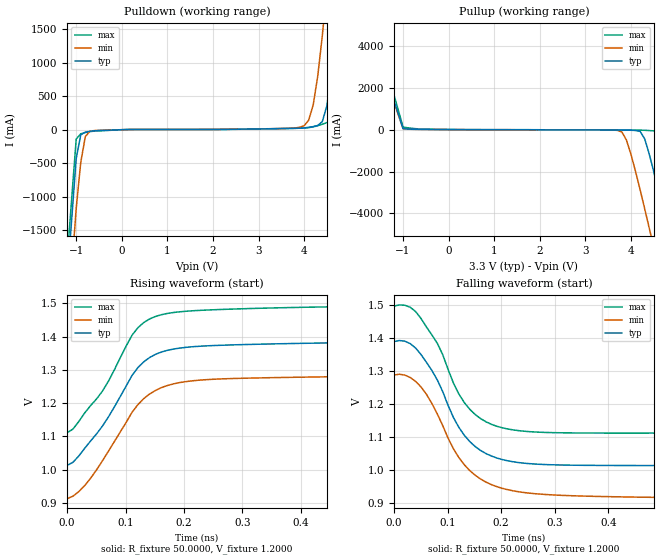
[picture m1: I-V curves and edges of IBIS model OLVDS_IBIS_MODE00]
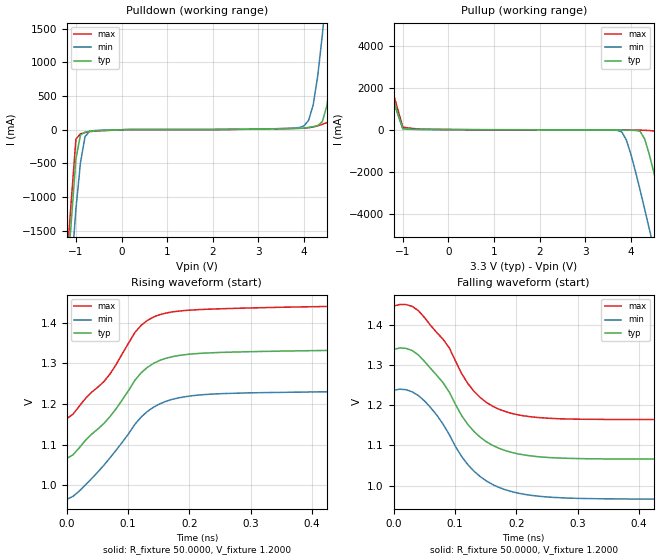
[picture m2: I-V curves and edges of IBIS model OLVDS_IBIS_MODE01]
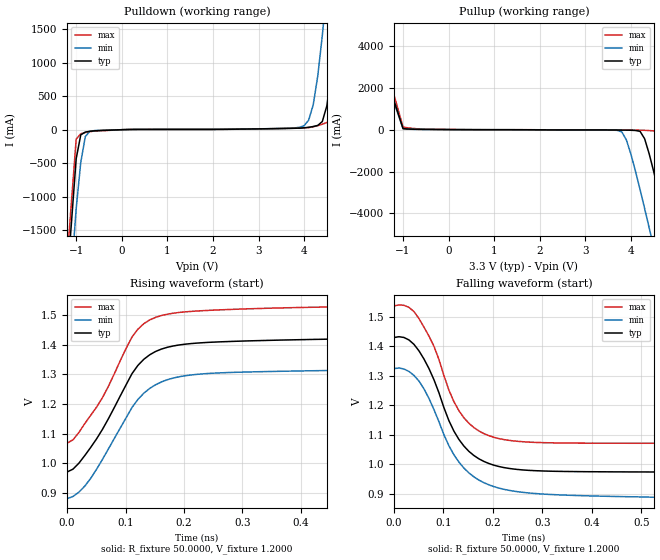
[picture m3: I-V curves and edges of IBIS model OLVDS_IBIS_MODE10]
| modified package RLC table on Oct 18th
| IBIS file olvds_ibis.ibs created by s2ibis2 version 1.1
| North Carolina State University Electronics Research Laboratory  1995
[IBIS ver]   3.2
[File name]   olvds_ibis.ibs
[File Rev]   1.0
[Date]   Oct 18, 2004
[Source]   Data created at Wipro Technologies
[Notes]   GS30 LVDS Driver
[Disclaimer] Please be aware that in the absence of a written agreement,
   Texas Instruments (TI) assumes no liability for: 1) the
   accuracy of the IBIS models provided to your company, 2) the
   proper functioning of these IBIS models in your design or for
   any resulting applications, or; 3) infringement of patents,
   copyrights, or intellectual property rights resulting from
   your use of these IBIS models. TI provides IBIS models as a
   service to our customers and therefore reserves the right to
   limit distribution of the IBIS models.
[Copyright]   Property of Texas Instruments Incorporated. Unauthorized
   reproduction and/or distribution is strictly prohibited. This
   product is protected under copyright law and trade secret law
   as an unpublished work. Copyright (C) 2003, Texas Instruments
   Incorporated, all rights reserved. These commodities are under
   the U.S. Government distribution license control. As such,
   they are not to be re-exported without the prior approval of
   the U.S. Department of Commerce.
|   Component OLVDS_IBIS
[Component]   OLVDS_IBIS
[Manufacturer]   Texas Instruments.
[Package]
| variable   typ   min   max
R_pkg   0.2   0.2   0.2
L_pkg   3.1nH   1.5nH   5.0nH
C_pkg   2.4pF   1.8pF   3.1pF
[Pin]  signal_name   model_name   R_pin   L_pin   C_pin
1   AVDD   POWER
|2   INP1   dummy
|3   INM1   dummy
4   AVSS   GND
|5   INP2   dummy
|6   INM2   dummy
7   AVDD   POWER
8   AVSS   GND
|9   INP3   dummy
|10   INM3   dummy
11   AVSS   GND
|12   INP4   dummy
|13   INM4   dummy
14   AVDD   POWER
15   LVSS   GND
|16   PD   dummy
17   LVSS   GND
18   LVSS   GND
19   LCLKP   OPERATIONAL_MODE
20   LCLKM   OPERATIONAL_MODE
21   OUTP1   OPERATIONAL_MODE
22   OUTM1   OPERATIONAL_MODE
23   OUTP2   OPERATIONAL_MODE
24   OUTM2   OPERATIONAL_MODE
25   LVDD   POWER
26   LVSS   GND
27   OUTP3   OPERATIONAL_MODE
28   OUTM3   OPERATIONAL_MODE
29   OUTP4   OPERATIONAL_MODE
30   OUTM4   OPERATIONAL_MODE
31   OUTP5   OPERATIONAL_MODE
32   OUTM5   OPERATIONAL_MODE
33   OUTP6   OPERATIONAL_MODE
34   OUTM6   OPERATIONAL_MODE
35   LVDD   POWER
36   LVSS   GND
37   OUTP7   OPERATIONAL_MODE
38   OUTM7   OPERATIONAL_MODE
39   OUTP8   OPERATIONAL_MODE
40   OUTM8   OPERATIONAL_MODE
41   ADCLKP   OPERATIONAL_MODE
42   ADCLKM   OPERATIONAL_MODE
43   LVSS   GND
44   LVSS   GND
|45   RESETZ   dummy
46   LVSS   GND
47   AVDD   POWER
|48   INP5   dummy
|49   INM5   dummy
50   AVSS   GND
|51   INP6   dummy
|52   INM6   dummy
53   AVSS   GND
54   AVDD   POWER
|55   INP7   dummy
|56   INM7   dummy
57   AVSS   GND
|58   INP8   dummy
|59   INM8   dummy
60   AVDD   POWER
61   AVSS   GND
62   AVSS   GND
63   AVDD   POWER
|64   ISET   dummy
|65   VCM   dummy
|66   REFM   dummy
|67   REFP   dummy
68   AVSS   GND
|69   INT   dummy
70   AVDD   POWER
|71   ADCLK   dummy
72   AVSS   GND
73   AVSS   GND
74   AVSS   GND
75   AVDD   POWER
|76   CSZ   dummy
|77   SDA   dummy
|78   SCLK   dummy
79   AVSS   GND
80   AVSS   GND
[Diff Pin]   inv_pin   vdiff   tdelay_typ   tdelay_min   tdelay_max
19   20   350mV   0   0   0
21   22   350mV   0   0   0
23   24   350mV   0   0   0
27   28   350mV   0   0   0
29   30   350mV   0   0   0
31   32   350mV   0   0   0
33   34   350mV   0   0   0
37   38   350mV   0   0   0
39   40   350mV   0   0   0
41   42   350mV   0   0   0
[Model Selector]   OPERATIONAL_MODE
OLVDS_IBIS_MODE00   Cell with  current setting of 3.5mA
OLVDS_IBIS_MODE01   Cell with  current setting of 2.5mA
OLVDS_IBIS_MODE10   Cell with  current setting of 4.5mA
OLVDS_IBIS_MODE11   Cell with  current setting of 6.0mA
| Models and submodels in the file (4): OLVDS_IBIS_MODE00 (Output), OLVDS_IBIS_MODE01 (Output), OLVDS_IBIS_MODE10 (Output), OLVDS_IBIS_MODE11 (Output)
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|   Model OLVDS_IBIS_MODE00
[Model]   OLVDS_IBIS_MODE00
Model_type   Output
Polarity   Inverting
Vmeas =   1.2000V
Cref =   5.0000pF
Rref = 50.0000
Vref =   1.2000V
C_comp   2.0000pF   1.5000pF   2.5000pF
[Temperature Range]   25.0000   0.1250k   -40.0000
[Voltage Range]   3.3000V   3.0000V   3.6000V
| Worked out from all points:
|   slope of the pulldown table from 0 to 0.495 V, typ, clamps not added: 131 ohm
|   slope of the pullup table from 0 to 0.495 V, typ, clamps not added: 106 ohm
|   rising waveform, R_fixture 50.0000, V_fixture 1.2000: 20-80 % time 83.5ps typ, 84.2ps min, 79.4ps max; typ from 1.01 V to 1.39 V
|   falling waveform, R_fixture 50.0000, V_fixture 1.2000: 20-80 % time 74.4ps typ, 82.1ps min, 72.4ps max; typ from 1.39 V to 1.01 V
[Pulldown]
| voltage   I(typ)   I(min)   I(max)
-3.3V     -22.38A    -23.14A    -21.96A
-2V       -9.6A      -10.42A    -9.138A
-1V       -431.5mA   -1.175A    -140.1mA
-900mV    -77.67mA   -488.8mA   -60.72mA
-800mV    -35.24mA   -102.6mA   -42.54mA
4V        27.23mA    59.11mA    24.41mA
4.2V      46.48mA    369mA      42.24mA
4.4V      121mA      1.402A     81.02mA
4.5V      356.5mA    2.114A     106.7mA
4.7V      1.539A     3.721A     310.2mA
4.9V      3.159A     5.456A     1.534A
6.6V      19.22A     21.51A     17.53A
[Pullup]
| voltage   I(typ)   I(min)   I(max)
-3.3V     19.22A     18.61A     20.47A
-2V       6.763A     6.35A      7.855A
-1V       50.05mA    51.47mA    127mA
3.8V      -16.47mA   -107.5mA   -13.35mA
4V        -25.62mA   -1.176A    -16.52mA
4.3V      -431.6mA   -3.769A    -27.64mA
4.4V      -1.156A    -4.693A    -40.05mA
4.6V      -2.911A    -6.576A    -136.4mA
4.8V      -4.781A    -8.488A    -1.51A
5.1V      -7.659A    -11.39A    -4.292A
5.2V      -8.628A    -12.36A    -5.251A
6.6V      -22.38A    -26.1A     -18.99A
[Ramp]
| variable   typ   min   max
dV/dt_r   0.2246/82.6494p   0.2234/83.4154p   0.2303/78.5899p
dV/dt_f   0.2250/73.6988p   0.2245/81.2654p   0.2302/71.7003p
R_load = 50.0000
[Rising Waveform]
R_fixture = 50.0000
V_fixture = 1.2000
V_fixture_min = 1.1000
V_fixture_max = 1.3000
| time   V(typ)   V(min)   V(max)
0s        1.013V     913.1mV    1.111V
10.1ps    1.022V     920.6mV    1.122V
30.3ps    1.065V     952.9mV    1.171V
60.61ps   1.131V     1.027V     1.236V
111.1ps   1.283V     1.172V     1.404V
121.2ps   1.307V     1.196V     1.427V
161.6ps   1.354V     1.247V     1.466V
212.1ps   1.369V     1.267V     1.477V
292.9ps   1.375V     1.274V     1.483V
1ns       1.387V     1.285V     1.495V
[Falling Waveform]
R_fixture = 50.0000
V_fixture = 1.2000
V_fixture_min = 1.1000
V_fixture_max = 1.3000
| time   V(typ)   V(min)   V(max)
0s        1.39V      1.288V     1.497V
20.2ps    1.391V     1.288V     1.5V
40.4ps    1.37V      1.269V     1.481V
80.81ps   1.274V     1.171V     1.385V
111.1ps   1.159V     1.065V     1.264V
131.3ps   1.106V     1.017V     1.205V
161.6ps   1.06V      973.8mV    1.157V
202ps     1.033V     945.6mV    1.129V
383.8ps   1.015V     920.9mV    1.113V
1ns       1.015V     914.2mV    1.113V
|   Model OLVDS_IBIS_MODE01
[Model]   OLVDS_IBIS_MODE01
Model_type   Output
Polarity   Inverting
Vmeas =   1.2000V
Cref =   5.0000pF
Rref = 50.000
Vref =   1.2000V
C_comp   2.0000pF   1.5000pF   2.5000pF
[Temperature Range]   25.0000   0.1250k   -40.0000
[Voltage Range]   3.3000V   3.0000V   3.6000V
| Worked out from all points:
|   slope of the pulldown table from 0 to 0.495 V, typ, clamps not added: 183 ohm
|   slope of the pullup table from 0 to 0.495 V, typ, clamps not added: 106 ohm
|   rising waveform, R_fixture 50.0000, V_fixture 1.2000: 20-80 % time 88.9ps typ, 88.6ps min, 83.5ps max; typ from 1.07 V to 1.34 V
|   falling waveform, R_fixture 50.0000, V_fixture 1.2000: 20-80 % time 76.3ps typ, 76.9ps min, 74.5ps max; typ from 1.34 V to 1.07 V
[Pulldown]
| voltage   I(typ)   I(min)   I(max)
-3.3V     -22.38A    -23.14A    -21.96A
-2V       -9.6A      -10.42A    -9.138A
-1V       -431.5mA   -1.175A    -140.1mA
-900mV    -77.58mA   -488.7mA   -60.61mA
-800mV    -35.11mA   -102.5mA   -42.41mA
4V        26.09mA    57.99mA    23.27mA
4.2V      45.33mA    368.2mA    41.09mA
4.4V      119.9mA    1.402A     79.85mA
4.5V      355.7mA    2.114A     105.5mA
4.7V      1.539A     3.721A     309.3mA
4.9V      3.159A     5.456A     1.534A
6.6V      19.22A     21.51A     17.53A
[Pullup]
| voltage   I(typ)   I(min)   I(max)
-3.3V     19.22A     18.61A     20.47A
-2V       6.763A     6.35A      7.855A
-1V       50.02mA    51.46mA    127mA
3.8V      -15.23mA   -106mA     -12.14mA
4V        -24.39mA   -1.176A    -15.32mA
4.3V      -430.8mA   -3.769A    -26.45mA
4.4V      -1.156A    -4.693A    -38.86mA
4.6V      -2.91A     -6.576A    -135.1mA
4.8V      -4.781A    -8.488A    -1.51A
5.1V      -7.659A    -11.39A    -4.292A
5.2V      -8.628A    -12.36A    -5.251A
6.6V      -22.38A    -26.1A     -18.99A
[Ramp]
| variable   typ   min   max
dV/dt_r   0.1623/88.0272p   0.1614/87.7741p   0.1681/82.6634p
dV/dt_f   0.1629/75.4883p   0.1623/76.1054p   0.1682/73.8001p
R_load = 50.0000
[Rising Waveform]
R_fixture = 50.0000
V_fixture = 1.2000
V_fixture_min = 1.1000
V_fixture_max = 1.3000
| time   V(typ)   V(min)   V(max)
0s        1.066V     965.8mV    1.164V
20.2ps    1.092V     985.8mV    1.194V
70.71ps   1.169V     1.068V     1.274V
111.1ps   1.258V     1.15V      1.376V
121.2ps   1.276V     1.168V     1.393V
141.4ps   1.3V       1.192V     1.414V
161.6ps   1.312V     1.206V     1.423V
212.1ps   1.324V     1.222V     1.432V
292.9ps   1.328V     1.227V     1.436V
1ns       1.337V     1.235V     1.444V
[Falling Waveform]
R_fixture = 50.0000
V_fixture = 1.2000
V_fixture_min = 1.1000
V_fixture_max = 1.3000
| time   V(typ)   V(min)   V(max)
0s        1.339V     1.237V     1.446V
20.2ps    1.341V     1.238V     1.45V
40.4ps    1.325V     1.224V     1.434V
90.91ps   1.232V     1.127V     1.342V
111.1ps   1.174V     1.072V     1.278V
131.3ps   1.134V     1.036V     1.234V
161.6ps   1.1V       1.003V     1.197V
202ps     1.079V     982.1mV    1.176V
343.4ps   1.067V     967.7mV    1.165V
1ns       1.067V     966.5mV    1.166V
|   Model OLVDS_IBIS_MODE10
[Model]   OLVDS_IBIS_MODE10
Model_type   Output
Polarity   Inverting
Vmeas =   1.2000V
Cref =   5.0000pF
Rref = 50.000
Vref =   1.2000V
C_comp   2.0000pF   1.5000pF   2.5000pF
[Temperature Range]   25.0000   0.1250k   -40.0000
[Voltage Range]   3.3000V   3.0000V   3.6000V
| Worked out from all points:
|   slope of the pulldown table from 0 to 0.495 V, typ, clamps not added: 107 ohm
|   slope of the pullup table from 0 to 0.495 V, typ, clamps not added: 107 ohm
|   rising waveform, R_fixture 50.0000, V_fixture 1.2000: 20-80 % time 80.4ps typ, 82.7ps min, 76.7ps max; typ from 0.97 V to 1.43 V
|   falling waveform, R_fixture 50.0000, V_fixture 1.2000: 20-80 % time 73.6ps typ, 84.3ps min, 70.9ps max; typ from 1.43 V to 0.973 V
[Pulldown]
| voltage   I(typ)   I(min)   I(max)
-3.3V     -22.38A    -23.14A    -21.96A
-2V       -9.6A      -10.42A    -9.138A
-1V       -431.6mA   -1.175A    -140.2mA
-900mV    -77.73mA   -488.9mA   -60.78mA
-800mV    -35.32mA   -102.7mA   -42.61mA
4V        28.14mA    59.96mA    25.34mA
4.2V      47.41mA    369.6mA    43.19mA
4.4V      121.8mA    1.403A     81.98mA
4.5V      357.1mA    2.115A     107.7mA
4.7V      1.539A     3.721A     310.8mA
4.9V      3.16A      5.456A     1.534A
6.6V      19.22A     21.51A     17.53A
[Pullup]
| voltage   I(typ)   I(min)   I(max)
-3.3V     19.22A     18.61A     20.47A
-2V       6.763A     6.35A      7.855A
-1V       50.06mA    51.48mA    127.1mA
3.8V      -17.4mA    -108.6mA   -14.26mA
4V        -26.6mA    -1.177A    -17.43mA
4.3V      -432.2mA   -3.769A    -28.54mA
4.4V      -1.156A    -4.693A    -40.95mA
4.6V      -2.911A    -6.576A    -137.5mA
4.8V      -4.781A    -8.488A    -1.51A
5.1V      -7.659A    -11.39A    -4.292A
5.2V      -8.628A    -12.36A    -5.251A
6.6V      -22.38A    -26.1A     -18.99A
[Ramp]
| variable   typ   min   max
dV/dt_r   0.2741/79.6048p   0.2646/81.8906p   0.2804/75.9843p
dV/dt_f   0.2744/72.9013p   0.2652/83.4654p   0.2802/70.2139p
R_load = 50.0000
[Rising Waveform]
R_fixture = 50.0000
V_fixture = 1.2000
V_fixture_min = 1.1000
V_fixture_max = 1.3000
| time   V(typ)   V(min)   V(max)
0s        970.4mV    880.1mV    1.068V
10.1ps    980mV      887.6mV    1.079V
40.4ps    1.054V     948.8mV    1.162V
60.61ps   1.115V     1.013V     1.222V
111.1ps   1.303V     1.189V     1.427V
131.3ps   1.351V     1.237V     1.472V
161.6ps   1.386V     1.275V     1.499V
212.1ps   1.404V     1.298V     1.513V
292.9ps   1.413V     1.308V     1.521V
1ns       1.427V     1.321V     1.535V
[Falling Waveform]
R_fixture = 50.0000
V_fixture = 1.2000
V_fixture_min = 1.1000
V_fixture_max = 1.3000
| time   V(typ)   V(min)   V(max)
0s        1.43V      1.325V     1.538V
40.4ps    1.407V     1.302V     1.518V
60.61ps   1.357V     1.256V     1.466V
80.81ps   1.287V     1.186V     1.401V
111.1ps   1.148V     1.062V     1.251V
131.3ps   1.084V     1.007V     1.182V
161.6ps   1.029V     956.8mV    1.124V
202ps     996.4mV    923.5mV    1.091V
363.6ps   974.7mV    893.6mV    1.071V
1ns       972.9mV    882.5mV    1.071V
